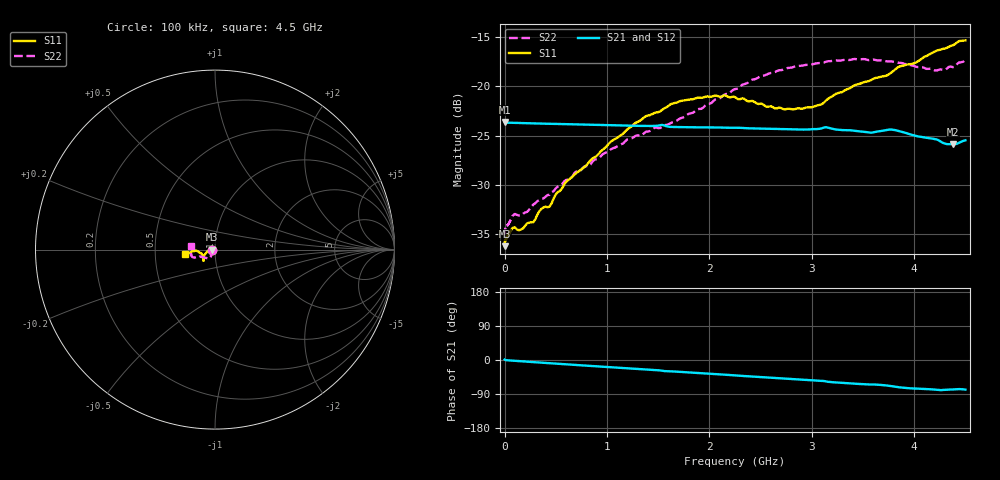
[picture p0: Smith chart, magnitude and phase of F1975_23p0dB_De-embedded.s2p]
! Integrated Device Technology
! Corporate Headquarters
! 6024 Silver Creek Valley Road
! San Jose, CA 95138  USA
! Phone:  1-408-284-8200
! Toll Free:  1-800-223-1366
! Webpage:  http://www.idt.com/
! Timing and RF Division
! 515 Groton Road, Suite 102
! Westford, MA 01886-6024
! Device:  F1975
! Description: 6-bit, 75 ohm, 0.5 dB Digital Step Attenuator
! Frequency:  5.0 MHz -  3.00 GHz
! Package:  4x4 mm QFN Plastic Package: 20 pin
! Ports:  2 RF, 11 DC
!  Pin  1  = D5 (16 dB)
!  Pin  2  = RF1  =  Port 1
!  Pin  3  = Serial Data In (DATA)
!  Pin  4  = Serial Clock (CLK)
!  Pin  5  = Serial Latch Enable (LE)
!  Pin  6  = VDD
!  Pin  7  = NC
!  Pin  8  = NC
!  Pin  9  = NC
!  Pin 10  = GND
!  Pin 11  = GND
!  Pin 12  = NC
!  Pin 13  = VMODE
!  Pin 14  = RF2  =  Port 2
!  Pin 15  = D4 (8 dB)
!  Pin 16  = D3 (4 dB)
!  Pin 17  = D2 (2 dB)
!  Pin 18  = NC
!  Pin 19  = D1 (1 dB)
!  Pin 20  = D0 (0.5 dB)
! State:  46
! Atten State:  23.0 dB
! Voltage:  +3.30 Volts
! Current:  0.597 mA
! Data:  The device was measured on a F1975 evaluation board which has
!  individual transmission lines to the RF pins.  Data was collected
!  using a calibrated network analyzer.  The evaluation board was
!  de-embedded using Automatic Fixture Removal (AFR).
!  The reference plane is the edge of the package pin.
! Misc:
!  Action Tracker AT0415
! Date Measured:  2018-02-08
! Date:  2018-03-26  MJV
! Note:
!  Integrated Device Technology supplies this data as a sample of measured
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# GHz S dB R 75
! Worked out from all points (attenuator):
!   291 points, 100 kHz to 4.5 GHz, reference 75 ohm
!   highest |S21| = -23.62 dB at 100 kHz (marker M1); lowest = -25.9 dB at 4.38 GHz (marker M2)
!   lowest |S11| = -36.2 dB at 100 kHz (marker M3), VSWR 1.03, Z = 72.7 + j0.000388 ohm
!   |S11| at or under -10 dB: start of sweep to end of sweep
!   |S22| runs from -35.1 to -17.2 dB; largest |S21 - S12| = 0.00016
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0.0001  -36.22 180.0  -23.62 1.2  -23.62 1.3  -35.08 -178.9
0.003  -35.71 -178.6  -23.67 0.7  -23.66 0.7  -34.61 -177.6
0.011  -35.51 -178.1  -23.69 -0.4  -23.69 -0.4  -34.30 -175.7
0.08  -34.37 -176.3  -23.71 -1.7  -23.71 -1.7  -33.12 -166.1
0.16  -34.51 -177.7  -23.74 -3.3  -23.74 -3.3  -33.11 -154.1
0.28  -33.79 179.4  -23.77 -5.5  -23.77 -5.5  -32.00 -144.5
0.36  -32.43 179.6  -23.79 -7.0  -23.79 -7.0  -31.42 -136.8
0.44  -32.19 -179.8  -23.81 -8.5  -23.81 -8.5  -31.02 -131.1
0.6  -29.70 -176.2  -23.85 -11.4  -23.85 -11.4  -29.50 -126.3
0.76  -28.35 -169.4  -23.89 -14.3  -23.89 -14.3  -28.32 -123.5
1.28  -23.71 -152.9  -24.01 -23.4  -24.01 -23.4  -25.03 -123.0
1.52  -22.55 -145.6  -23.95 -27.5  -23.95 -27.5  -24.24 -129.5
1.64  -21.76 -142.8  -24.13 -30.1  -24.13 -30.1  -23.65 -133.4
1.88  -21.18 -138.7  -24.18 -34.0  -24.17 -34.0  -22.36 -144.4
2.26  -21.17 -137.2  -24.22 -40.8  -24.21 -40.7  -20.27 -155.3
2.64  -22.25 -147.5  -24.33 -47.4  -24.32 -47.4  -18.57 -158.4
3.02  -22.08 -164.2  -24.35 -53.7  -24.35 -53.7  -17.75 -160.8
3.42  -19.90 -175.7  -24.53 -62.6  -24.52 -62.6  -17.24 -166.3
3.76  -18.75 -175.8  -24.40 -68.4  -24.39 -68.4  -17.49 -172.7
4.2  -16.49 -172.5  -25.36 -78.1  -25.36 -78.1  -18.40 175.5
4.38  -15.85 -170.2  -25.89 -77.7  -25.88 -77.7  -18.07 173.2
4.5  -15.36 -171.7  -25.48 -78.2  -25.48 -78.2  -17.31 170.6
